(* Logix 5000 AddOnInstructionDefinition export wxsHeartbeat_DataLogger; software revision 32.00 *)

ADD_ON_INSTRUCTION wxsHeartbeat_DataLogger   (* revision 1.0, vendor Pendant Automation *)
// Heartbeat AOI for Data Logger and other Misc. Middleware Features
VAR_INPUT
   TimeoutSetpoint : DINT; {required}
   TxHeartbeat : BOOL; {required}
END_VAR
VAR_OUTPUT
   LossOfComms : BOOL; {access Read Only, visible}
END_VAR
VAR
   tmrHeartbeat_True : TIMER; {access None}
   tmrHeartbeat_False : TIMER; {access None}
END_VAR

ROUTINE Logic   (* ladder *)
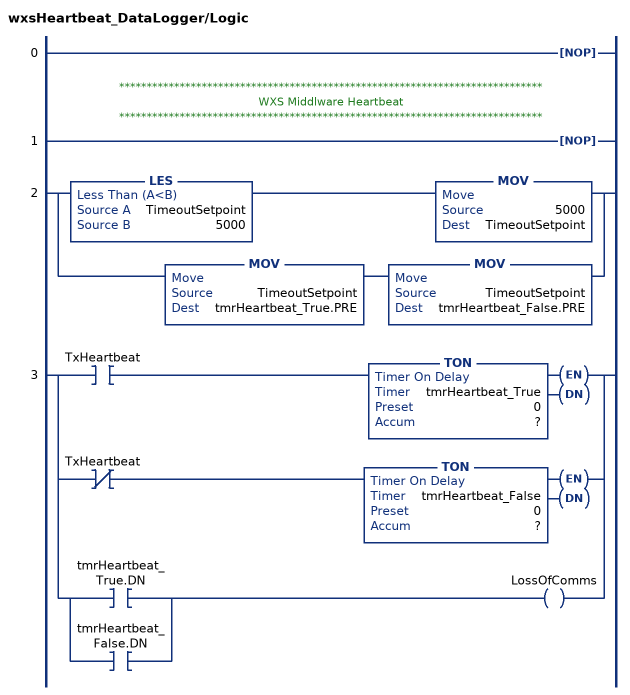
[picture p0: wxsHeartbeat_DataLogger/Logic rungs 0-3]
   0: NOP();
   // *****************************************************************************
   // WXS Middlware Heartbeat
   // *****************************************************************************
   1: NOP();
   2: [LES(TimeoutSetpoint,5000) MOV(5000,TimeoutSetpoint) ,MOV(TimeoutSetpoint,tmrHeartbeat_True.PRE) MOV(TimeoutSetpoint,tmrHeartbeat_False.PRE) ];
   3: [XIC(TxHeartbeat) TON(tmrHeartbeat_True,?,?) ,XIO(TxHeartbeat) TON(tmrHeartbeat_False,?,?) ,[XIC(tmrHeartbeat_True.DN) ,XIC(tmrHeartbeat_False.DN) ] OTE(LossOfComms) ];
END_ROUTINE
END_ADD_ON_INSTRUCTION
